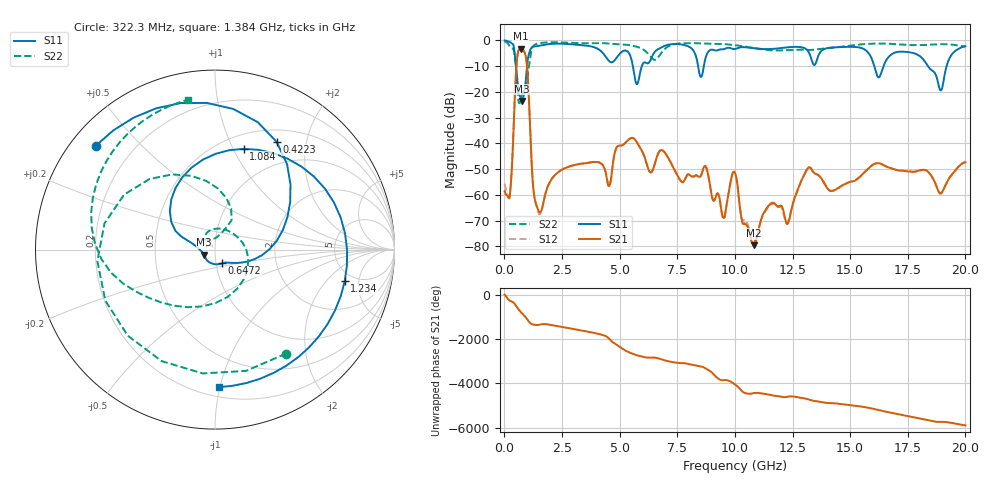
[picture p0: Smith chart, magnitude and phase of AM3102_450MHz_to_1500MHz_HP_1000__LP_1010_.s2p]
!Agilent Technologies,E8364B,MY43040894,A.07.50.67
!Agilent E8364B: A.07.50.67
!Date: Thursday, January 11, 2018 05:58:57
!Correction: S11(Full 2 Port(1,2))
!S21(Full 2 Port(1,2))
!S12(Full 2 Port(1,2))
!S22(Full 2 Port(1,2))
!S2P File: Measurements: S11, S21, S12, S22:
# Hz S  dB  R 50
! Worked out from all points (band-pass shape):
!   1601 points, 10 MHz to 20 GHz, reference 50 ohm
!   highest |S21| = -3.28 dB at 709.6 MHz (marker M1); lowest = -79.5 dB at 10.84 GHz (marker M2)
!   |S21| within 3 dB of the highest: 561.6 MHz to 928.2 MHz (366.6 MHz wide, 49.2 % of centre)
!   lowest |S11| = -23.5 dB at 772.1 MHz (marker M3), VSWR 1.14, Z = 44.2 - j2.54 ohm
!   |S11| at or under -10 dB: 506.2 MHz to 980.1 MHz (473.9 MHz wide, 63.8 % of centre); 16.05 GHz to 16.45 GHz (403.6 MHz wide, 2.48 % of centre); 18.37 GHz to 19.18 GHz (813.5 MHz wide, 4.33 % of centre)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
!   |S22| runs from -24.4 to -0.4 dB; largest |S21 - S12| = 0.00092
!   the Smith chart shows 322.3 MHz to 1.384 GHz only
!   S11 on the Smith chart (normalised r, x): 322.3 MHz: 0.07, +0.37; 422.3 MHz: 0.66, +1.52; 647.2 MHz: 1.07, -0.16; 1.084 GHz: 0.65, +1.10; 1.234 GHz: 4.14, -3.27; 1.384 GHz: 0.27, -0.99
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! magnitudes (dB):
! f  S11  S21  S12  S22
! 10 MHz  -0.1  -58.5  -55.6  -0.4
! 322.3 MHz  -1.1  -50.0  -49.6  -3.1
! 422.3 MHz  -3.2  -28.2  -28.1  -4.6
! 647.2 MHz  -21.3  -3.5  -3.5  -24.4
! 709.6 MHz  -22.2  -3.3  -3.3  -23.8
! 772.1 MHz  -23.5  -3.4  -3.4  -20.6
! 1.084 GHz  -4.7  -26.8  -26.8  -9.0
! 1.234 GHz  -2.6  -55.4  -55.3  -2.4
! 1.384 GHz  -2.3  -63.8  -64.0  -1.4
! 3.346 GHz  -1.9  -47.8  -47.8  -1.1
! 4.545 GHz  -8.1  -56.5  -56.4  -1.2
! 4.895 GHz  -6.5  -41.2  -41.2  -1.5
! 5.745 GHz  -17.0  -39.5  -39.5  -2.5
! 6.682 GHz  -3.4  -43.7  -43.7  -6.5
! 8.731 GHz  -6.8  -48.9  -48.9  -1.2
! 9.505 GHz  -3.5  -68.9  -69.1  -1.5
! 10.01 GHz  -3.4  -51.5  -51.5  -1.9
! 10.84 GHz  -3.1  -79.5  -79.6  -3.1
! 13.34 GHz  -8.0  -50.2  -50.2  -3.7
! 16.68 GHz  -6.4  -49.4  -49.3  -1.3
! 18.93 GHz  -19.4  -59.4  -59.6  -1.5
! 20 GHz  -2.3  -47.3  -47.1  -2.4
